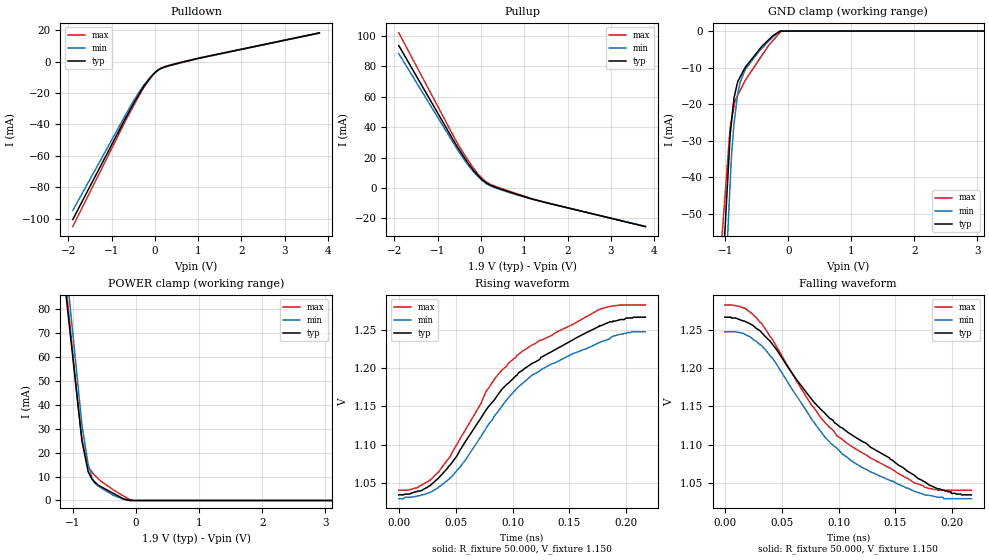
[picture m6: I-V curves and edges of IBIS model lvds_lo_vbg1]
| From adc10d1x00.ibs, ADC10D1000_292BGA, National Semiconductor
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[Model]   lvds_lo_vbg1
Model_type Output
Vref=1.150E+00
Rref=5.000E+01
Cref=0.000E+00
Vmeas=1.150E+00
C_comp   4.84E-13   4.84E-13   4.84E-13
[Voltage Range]   1.900E+00   1.800E+00   2.000E+00
[POWER Clamp Reference]   1.900E+00   1.800E+00   2.000E+00
[GND Clamp Reference]   0.000E+00   0.000E+00   0.000E+00
[Pullup Reference]   1.900E+00   1.800E+00   2.000E+00
[Pulldown Reference]   0.000E+00   0.000E+00   0.000E+00
[Temperature Range]   25   85   -40
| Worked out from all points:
|   slope of the pulldown table from 0 to 0.285 V, typ, clamps not added: 68.3 ohm
|   slope of the pullup table from 0 to 0.285 V, typ, clamps not added: 55.7 ohm
|   GND clamp passes 1 mA (typ) near -0.22 V on its own axis
|   POWER clamp passes 1 mA (typ) near -0.22 V on its own axis
|   rising waveform, R_fixture 50.000, V_fixture 1.150: 20-80 % time 83.6ps typ, 77.3ps min, 75.3ps max; typ from 1.03 V to 1.27 V
|   falling waveform, R_fixture 50.000, V_fixture 1.150: 20-80 % time 98.5ps typ, 71.5ps min, 78.2ps max; typ from 1.27 V to 1.03 V
[GND Clamp]
-2V       -371mA     -429.8mA   -276.9mA
-1.8V     -307.6mA   -357.9mA   -230.5mA
-920mV    -28.36mA   -41.57mA   -26.18mA
-900mV    -25.04mA   -34.38mA   -24.38mA
-860mV    -18.4mA    -25.49mA   -20.78mA
-840mV    -16.88mA   -22.7mA    -18.98mA
-800mV    -13.83mA   -17.11mA   -17.61mA
-760mV    -12.53mA   -13.96mA   -16.23mA
-680mV    -9.914mA   -10.52mA   -13.48mA
-460mV    -5.124mA   -5.512mA   -7.792mA
-140mV    -206.8uA   0A         -590.3uA
4V        0A         0A         0A
[POWER Clamp]
-2.1V     324.3mA    359mA      348.3mA
-1.7V     227.7mA    253.4mA    243.6mA
-980mV    53.91mA    63.33mA    55.1mA
-920mV    39.43mA    47.49mA    39.39mA
-860mV    24.94mA    31.65mA    25.86mA
-760mV    11.91mA    14.93mA    14.12mA
-700mV    8.851mA    9.544mA    11.8mA
-660mV    7.856mA    7.285mA    10.54mA
-360mV    2.953mA    2.13mA     4.41mA
-200mV    678.3uA    486.8uA    1.865mA
-30mV     0A         0A         0A
3.9V      0A         0A         0A
[Pullup]
-1.9V     93.71mA    88.4mA     102.1mA
-640mV    31.57mA    29.78mA    34.4mA
-480mV    24.17mA    22.51mA    26.39mA
-320mV    17.25mA    15.93mA    19.22mA
-180mV    11.83mA    10.97mA    13.37mA
-60mV     7.921mA    7.266mA    9.004mA
120mV     3.435mA    2.994mA    4.167mA
380mV     120.7uA    -313.7uA   635.9uA
1.32V     -8.236mA   -8.303mA   -8.11mA
3.8V      -25.32mA   -25.19mA   -25.31mA
[Pulldown]
-1.9V     -100.4mA   -94.67mA   -104.9mA
-700mV    -36.99mA   -34.88mA   -38.67mA
-440mV    -24.06mA   -22.59mA   -25.25mA
-240mV    -15.13mA   -14.33mA   -15.74mA
-120mV    -10.7mA    -10.26mA   -11.04mA
40mV      -6.081mA   -5.928mA   -6.232mA
220mV     -3.415mA   -3.229mA   -3.609mA
600mV     -547.1uA   -354.4uA   -743.5uA
3.8V      18.24mA    18.32mA    18.13mA
[Rising Waveform]
R_fixture = 50.000
V_fixture = 1.150
V_fixture_min = 1.150
V_fixture_max = 1.150
|  time   V(typ)   V(min)   V(max)
0s        1.035V     1.03V      1.041V
15.75ps   1.039V     1.033V     1.044V
27.5ps    1.047V     1.038V     1.054V
46.75ps   1.077V     1.059V     1.09V
84.25ps   1.159V     1.138V     1.186V
108.7ps   1.197V     1.18V      1.222V
125ps     1.214V     1.198V     1.236V
177.8ps   1.255V     1.234V     1.277V
200.8ps   1.265V     1.246V     1.282V
216.8ps   1.266V     1.247V     1.282V
[Falling Waveform]
R_fixture = 50.000
V_fixture = 1.150
V_fixture_min = 1.150
V_fixture_max = 1.150
|  time   V(typ)   V(min)   V(max)
0s        1.266V     1.247V     1.282V
17.25ps   1.261V     1.244V     1.278V
31.75ps   1.247V     1.23V      1.259V
42.25ps   1.23V      1.212V     1.236V
76.5ps    1.159V     1.133V     1.151V
98.25ps   1.127V     1.096V     1.112V
120.2ps   1.105V     1.071V     1.09V
175.5ps   1.052V     1.035V     1.045V
199ps     1.037V     1.03V      1.041V
216.8ps   1.035V     1.03V      1.041V
[Ramp]
dV/dt_r   1.7620E+00/8.3690E-11   1.7024E+00/7.7090E-11   1.8230E+00/7.6220E-11
dV/dt_f   1.7620E+00/9.8602E-11   1.7024E+00/7.0687E-11   1.8230E+00/7.8609E-11
R_load = 50
